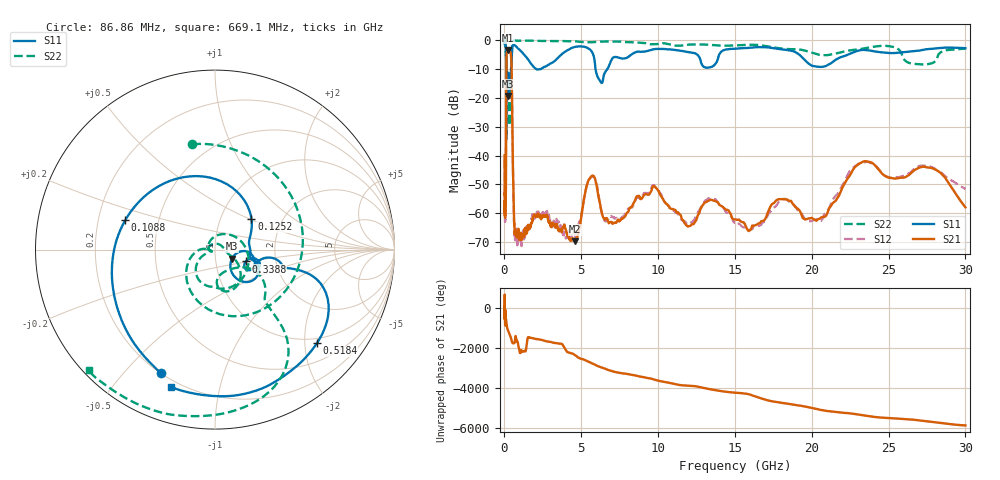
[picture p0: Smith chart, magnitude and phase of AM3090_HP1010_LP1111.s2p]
! Date/Time: Thu, Feb 28, 2019 2:05 PM
! Network Analyzer: Agilent Technologies E8364B Rev: A.07.50.67
! Sweep from 0.010 to 30.000 GHz, 1601 Points, Sweep Type: LOG
! Power Supply: 5.023 V, 0.002 A
# Hz S DB R 50
!freq MagS11 AngS11 MagS21 AngS21 MagS12 AngS12 MagS22 AngS22
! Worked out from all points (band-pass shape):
!   1601 points, 10 MHz to 30 GHz, reference 50 ohm
!   highest |S21| = -3.52 dB at 252.2 MHz (marker M1); lowest = -69.7 dB at 4.571 GHz (marker M2)
!   |S21| within 3 dB of the highest: 130 MHz to 442.7 MHz (312.6 MHz wide, 109 % of centre)
!   lowest |S11| = -19.4 dB at 244.7 MHz (marker M3), VSWR 1.24, Z = 60.1 - j6.14 ohm
!   |S11| at or under -10 dB: 122.4 MHz to 428.2 MHz (305.8 MHz wide, 111 % of centre); 2.035 GHz to 2.394 GHz (359.2 MHz wide, 16.2 % of centre); 5.926 GHz to 6.71 GHz (783.4 MHz wide, 12.4 % of centre)
!   |S22| runs from -34.3 to -0.2 dB; largest |S21 - S12| = 0.018
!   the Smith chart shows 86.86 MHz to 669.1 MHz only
!   S11 on the Smith chart (normalised r, x): 86.86 MHz: 0.20, -0.63; 108.8 MHz: 0.32, +0.14; 125.2 MHz: 1.40, +0.51; 338.8 MHz: 1.40, -0.19; 518.4 MHz: 0.89, -2.27; 669.1 MHz: 0.17, -0.72
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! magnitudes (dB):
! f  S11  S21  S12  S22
! 10 MHz  -0.3  -39.9  -41.4  -0.7
! 38.04 MHz  -0.5  -59.0  -58.2  -1.7
! 86.86 MHz  -2.5  -54.7  -53.3  -4.4
! 108.8 MHz  -5.6  -27.1  -27.0  -6.6
! 125.2 MHz  -11.5  -8.4  -8.4  -16.5
! 144.7 MHz  -14.0  -4.7  -4.7  -29.8
! 244.7 MHz  -19.4  -3.5  -3.5  -13.6
! 252.2 MHz  -18.7  -3.5  -3.5  -13.6
! 338.8 MHz  -14.7  -3.7  -3.7  -21.8
! 450.6 MHz  -8.0  -7.2  -7.2  -8.1
! 518.4 MHz  -2.3  -31.9  -31.9  -0.9
! 550.5 MHz  -1.9  -44.1  -43.5  -0.5
! 669.1 MHz  -1.9  -67.1  -67.9  -0.2
! 2.084 GHz  -10.2  -60.8  -59.9  -0.3
! 4.571 GHz  -2.5  -69.7  -68.4  -0.5
! 5.64 GHz  -3.7  -47.3  -47.6  -0.8
! 6.234 GHz  -14.3  -57.0  -57.5  -0.6
! 7.926 GHz  -6.3  -60.3  -59.4  -0.8
! 9.731 GHz  -3.2  -50.5  -50.3  -1.5
! 20.2 GHz  -9.2  -62.2  -62.3  -4.7
! 23.48 GHz  -3.5  -41.9  -42.3  -2.9
! 30 GHz  -2.9  -57.9  -51.6  -3.1
